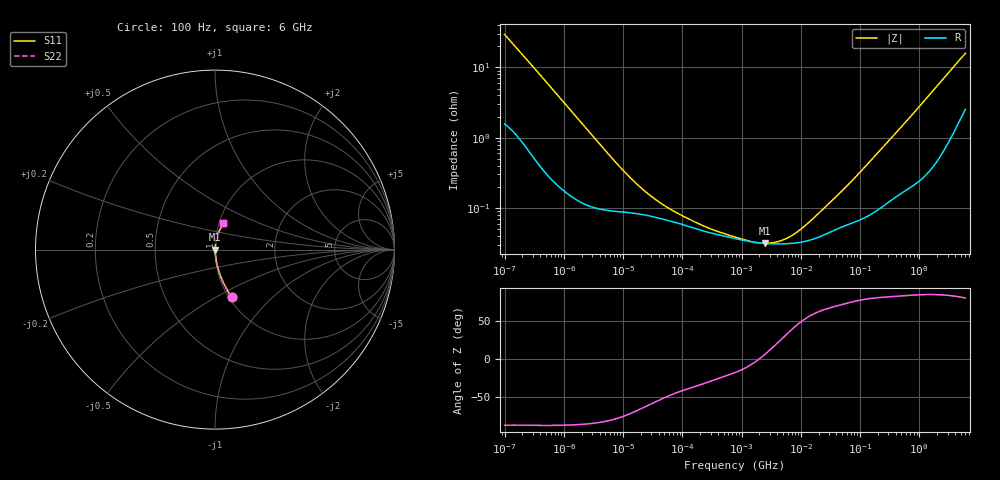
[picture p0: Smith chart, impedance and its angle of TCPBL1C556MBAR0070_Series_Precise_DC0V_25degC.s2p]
! TCPBL1C556MBAR0070 Polymer Tantalum Capacitor Sparameter Model
! Model Generated by Samsung Electro-Mechanics
! Samsung Sparameter Version 5.0
! Date : Oct-21-2025
! Products : Polymer Tantalum Capacitor
! Characteristics :
!  Nominal Capacitance = 55uF
!  Capacitance Tolerance = +/-20%
!  ESR = 70 mohm max at 100kHz
!  Rated Voltage = 16Vdc
!  Size = 1411(unit:inch), 3528(unit:mm)
!  Length = 3.50+/-0.20mm
!  Width = 2.80+/-0.20mm
!  Thickness = 1.90+/-0.10mm
!  Lineup = Conductive Polymer Type
!  Feature = PBL
!  Measurement Temperature : 25degC.
!  DC bias Value = 0V
!  Frequency : 100Hz ~ 6GHz
! External Node Assignments :
!  1  o---||---o  2
# MHz S RI R 50.0
! Freq.  Real(S11)  Im(S11)  Real(S12)  Im(S12)  Real(S21)  Im(S21)  Real(S22)  Im(S22)
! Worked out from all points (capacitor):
!   300 points, 100 Hz to 6 GHz, reference 50 ohm
!   read as one part in series: C = 53.3 uF near 106.2 Hz
!   lowest |Z| = 31.4 mohm at 2.491 MHz (marker M1)
!   series resonance near 1.953 MHz, so ESL is about 120 pH
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0.0001  0.0919 -0.2636  0.9081 0.2636  0.9081 0.2636  0.0919 -0.2636
0.0001820283  0.0356 -0.1593  0.9644 0.1593  0.9644 0.1593  0.0356 -0.1593
0.0003517965  0.0121 -0.0869  0.9879 0.0869  0.9879 0.0869  0.0121 -0.0869
0.0007664292  0.00381 -0.041  0.9962 0.041  0.9962 0.041  0.00381 -0.041
0.001998454  0.00144 -0.016  0.9986 0.016  0.9986 0.016  0.00144 -0.016
0.006236745  0.000935 -0.00523  0.9991 0.00523  0.9991 0.00523  0.000935 -0.00523
0.01205343  0.000866 -0.00278  0.9991 0.00278  0.9991 0.00278  0.000866 -0.00278
0.02194065  0.000803 -0.00162  0.9992 0.00162  0.9992 0.00162  0.000803 -0.00162
0.03993819  0.000717 -0.000991  0.9993 0.000991  0.9993 0.000991  0.000717 -0.000991
0.07718646  0.000619 -0.000608  0.9994 0.000608  0.9994 0.000608  0.000619 -0.000608
0.2012627  0.000484 -0.000322  0.9995 0.000322  0.9995 0.000322  0.000484 -0.000322
0.7981464  0.000365 -0.000113  0.9996 0.000113  0.9996 0.000113  0.000365 -0.000113
1.542536  0.000327 -3.24e-05  0.9997 3.24e-05  0.9997 3.24e-05  0.000327 -3.24e-05
2.490843  0.000312 3.62e-05  0.9997 -3.62e-05  0.9997 -3.62e-05  0.000312 3.62e-05
4.022142  0.000307 0.00012  0.9997 -0.00012  0.9997 -0.00012  0.000307 0.00012
6.117227  0.00031 0.000216  0.9997 -0.000216  0.9997 -0.000216  0.00031 0.000216
9.303617  0.000322 0.000349  0.9997 -0.000349  0.9997 -0.000349  0.000322 0.000349
15.95059  0.000359 0.000601  0.9996 -0.000601  0.9996 -0.000601  0.000359 0.000601
67.15989  0.000596 0.00218  0.9994 -0.00218  0.9994 -0.00218  0.000596 0.00218
318.7652  0.00133 0.00933  0.9987 -0.00933  0.9987 -0.00933  0.00133 0.00933
1810.813  0.00651 0.049  0.9935 -0.049  0.9935 -0.049  0.00651 0.049
6000  0.047 0.1457  0.953 -0.1457  0.953 -0.1457  0.047 0.1457
